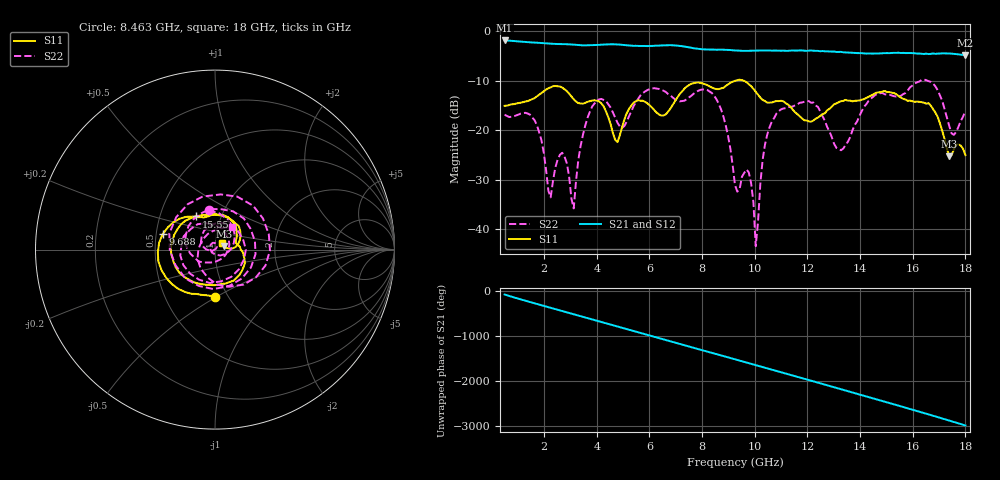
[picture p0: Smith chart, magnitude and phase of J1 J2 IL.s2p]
!Agilent Technologies,N5230A,MY45001360,A.07.50.67
!Agilent N5230A: A.07.50.67
!Date: Tuesday, April 16, 2024 16:20:41
!Correction: S11(Full 2 Port(1,2))
!S21(Full 2 Port(1,2))
!S12(Full 2 Port(1,2))
!S22(Full 2 Port(1,2))
!S2P File: Measurements: S11, S21, S12, S22:
# Hz S  dB  R 50
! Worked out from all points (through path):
!   201 points, 500 MHz to 18 GHz, reference 50 ohm
!   highest |S21| = -1.91 dB at 500 MHz (marker M1); lowest = -4.9 dB at 18 GHz (marker M2)
!   group delay of S21, straight-line fit = 460 ps
!   lowest |S11| = -25.3 dB at 17.39 GHz (marker M3), VSWR 1.12, Z = 55.3 + j2.19 ohm
!   |S11| at or under -10 dB: start of sweep to 9.289 GHz; 9.556 GHz to end of sweep
!   |S22| runs from -43.4 to -9.8 dB; largest |S21 - S12| = 0.0076
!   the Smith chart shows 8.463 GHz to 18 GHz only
!   S11 on the Smith chart (normalised r, x): 8.463 GHz: 0.87, -0.49; 9.688 GHz: 0.54, +0.10; 15.55 GHz: 0.76, +0.29; 18 GHz: 1.08, +0.08
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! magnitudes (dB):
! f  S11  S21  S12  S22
! 500 MHz  -15.1  -1.9  -1.9  -16.9
! 1.637 GHz  -13.6  -2.3  -2.3  -18.0
! 2.25 GHz  -11.4  -2.6  -2.6  -33.6
! 2.688 GHz  -11.4  -2.7  -2.7  -24.6
! 3.125 GHz  -13.8  -2.8  -2.7  -35.8
! 3.475 GHz  -14.7  -2.9  -2.9  -21.0
! 4.088 GHz  -14.2  -2.8  -2.8  -13.8
! 4.787 GHz  -22.4  -2.7  -2.7  -18.5
! 6.362 GHz  -16.9  -3.0  -2.9  -11.7
! 8.463 GHz  -11.6  -3.8  -3.8  -13.1
! 9.25 GHz  -10.1  -3.9  -3.9  -31.1
! 9.688 GHz  -10.3  -4.0  -4.0  -28.0
! 10.04 GHz  -12.3  -4.0  -4.0  -43.4
! 10.3 GHz  -13.9  -3.9  -3.9  -26.0
! 10.65 GHz  -14.4  -4.0  -4.0  -18.3
! 12.22 GHz  -18.1  -4.0  -4.0  -14.4
! 13.28 GHz  -14.2  -4.2  -4.3  -24.1
! 15.11 GHz  -12.3  -4.5  -4.4  -12.9
! 15.55 GHz  -13.4  -4.5  -4.4  -13.1
! 16.69 GHz  -15.1  -4.6  -4.6  -10.3
! 17.39 GHz  -25.3  -4.5  -4.6  -19.2
! 18 GHz  -25.1  -4.9  -4.9  -16.1
